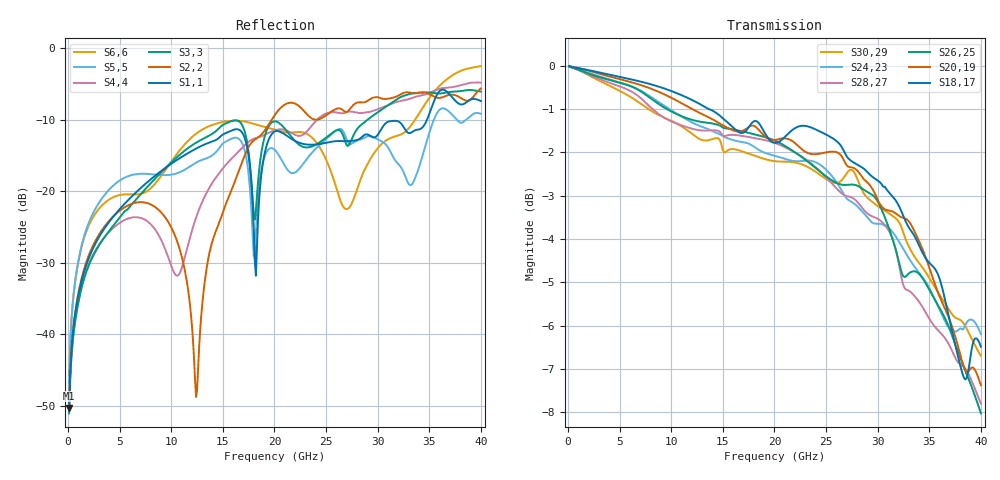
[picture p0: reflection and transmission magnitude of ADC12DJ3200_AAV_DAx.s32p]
! Touchstone file
! Texas Instruments 4/21/2021
! ADC12DJ2700AAV, ADC12DJ3200AAV, ADC08DJ3200AAV
! package type BGA
! High-speed serialized data output for channel A, lane 0-7
# GHZ S MA R 50.000000
! Port[1] = DA0N_BGA_F12
! Port[2] = DA0N_DIE_22
! Port[3] = DA0P_BGA_E12
! Port[4] = DA0P_DIE_21
! Port[5] = DA1N_BGA_D12
! Port[6] = DA1N_DIE_24
! Port[7] = DA1P_BGA_C12
! Port[8] = DA1P_DIE_23
! Port[9] = DA2N_BGA_A11
! Port[10] = DA2N_DIE_26
! Port[11] = DA2P_BGA_A10
! Port[12] = DA2P_DIE_25
! Port[13] = DA3N_BGA_A9
! Port[14] = DA3N_DIE_28
! Port[15] = DA3P_BGA_A8
! Port[16] = DA3P_DIE_27
! Port[17] = DA4N_BGA_F11
! Port[18] = DA4N_DIE_30
! Port[19] = DA4P_BGA_E11
! Port[20] = DA4P_DIE_29
! Port[21] = DA5N_BGA_D11
! Port[22] = DA5N_DIE_32
! Port[23] = DA5P_BGA_C11
! Port[24] = DA5P_DIE_31
! Port[25] = DA6N_BGA_B11
! Port[26] = DA6N_DIE_34
! Port[27] = DA6P_BGA_B10
! Port[28] = DA6P_DIE_33
! Port[29] = DA7N_BGA_B9
! Port[30] = DA7N_DIE_36
! Port[31] = DA7P_BGA_B8
! Port[32] = DA7P_DIE_35
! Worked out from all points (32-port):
!   400 points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, 100 MHz to 40 GHz, reference 50 ohm
!   strongest paths, dB at 100 MHz, 10.1 GHz, 20.1 GHz, 30.1 GHz, 40 GHz:
!     S18,17: 0.0, -0.6, -1.8, -2.7, -6.5
!     S20,19: 0.0, -0.8, -1.7, -3.1, -7.4
!     S26,25: 0.0, -1.1, -1.7, -3.2, -8.0
!     S28,27: 0.0, -1.3, -1.8, -3.5, -7.8
!     S24,23: 0.0, -1.0, -2.1, -3.6, -6.2
!     S30,29: 0.0, -1.3, -2.2, -3.3, -6.7
!   lowest |S11| = -50.3 dB at 100 MHz (marker M1), VSWR 1.01, Z = 50.2 + j0.259 ohm
!   |S11| at or under -10 dB: start of sweep to 34.78 GHz
